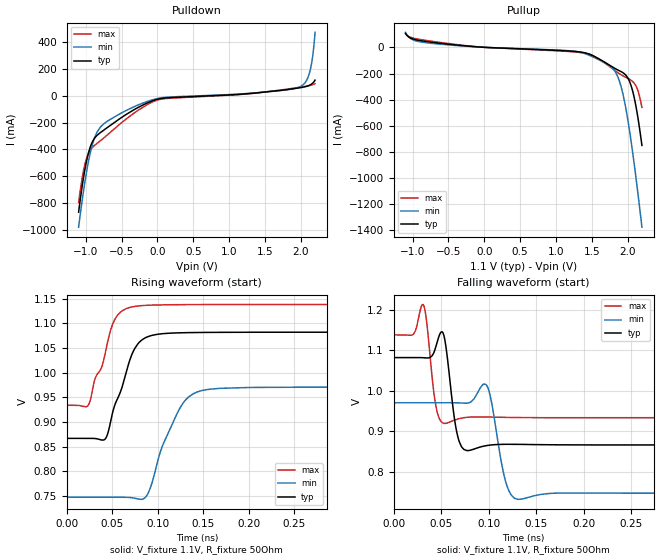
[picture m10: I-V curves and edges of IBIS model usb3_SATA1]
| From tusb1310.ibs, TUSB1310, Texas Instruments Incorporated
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|   USB 3.0 SATA1 mode, for SSTXP/N pin 750MHz
[Model]   usb3_SATA1
Model_type   Output
Polarity   Inverting
Vmeas = 0.96V
Vref = 1.1
Rref = 50
|   typ   min   max
|   (nom PVT)   (Fast PVT)   (slow PVT)
C_comp   0.5348pF   0.5225pF   0.5522pF
[Voltage Range]   1.1   0.99   1.155
[Temperature Range]   27   105   -40
[Pullup Reference]   1.1   0.99   1.155
[Pulldown Reference]   0   0   0
[Power Clamp Reference]   1.1   0.99   1.155
[GND Clamp Reference]   0   0   0
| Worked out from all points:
|   slope of the pulldown table from 0 to 0.165 V, typ, clamps not added: 14 ohm
|   slope of the pullup table from 0 to 0.165 V, typ, clamps not added: 40 ohm
|   falling waveform, V_fixture 1.1V, R_fixture 50Ohm: 20-80 % time 6.91ps typ, 9.83ps min, 5.71ps max; typ from 1.08 V to 0.867 V
|   rising waveform, V_fixture 1.1V, R_fixture 50Ohm: 20-80 % time 22.8ps typ, 27.8ps min, 20.9ps max; typ from 0.867 V to 1.08 V
[Pulldown]
|   Voltage   I(typ)   I(min)   I(max)
-1.1V     -868.9mA   -981.1mA   -796.9mA
-1.026V   -591.5mA   -690mA     -543.5mA
-951.1mV  -405.4mA   -461.1mA   -416.4mA
-868.4mV  -309.8mA   -301.2mA   -365.6mA
-744.4mV  -253.7mA   -206.5mA   -312.2mA
-297.7mV  -94.05mA   -73.91mA   -117.4mA
24.81mV   -21.49mA   -16.51mA   -26.68mA
1.977V    60.53mA    65.43mA    65.05mA
2.059V    68.81mA    98.55mA    72.03mA
2.117V    78.81mA    163.5mA    77.89mA
2.167V    95.9mA     297.7mA    84.86mA
2.2V      118.6mA    476.1mA    91.68mA
[Pullup]
|   Voltage   I(typ)   I(min)   I(max)
-1.1V     108.7mA    115.9mA    105.4mA
-992.5mV  63.95mA    57.32mA    71.65mA
-760.9mV  41.82mA    32.99mA    49.68mA
-16.54mV  1.455mA    1.316mA    1.593mA
1.406V    -41.39mA   -47.96mA   -43.61mA
1.77V     -143.3mA   -149.8mA   -155mA
1.877V    -176.7mA   -245mA     -198.4mA
1.968V    -208.9mA   -446.3mA   -227.1mA
2.026V    -260.1mA   -635.7mA   -243.8mA
2.084V    -364.9mA   -860.9mA   -269.2mA
2.142V    -532.4mA   -1.111A    -328.4mA
2.2V      -751.7mA   -1.378A    -460mA
[Ramp]
R_load = 50
|   typ   min   max
dV/dt_r   0.129193/2.27921e-11   0.134045/2.77619e-11   0.1226/2.09021e-11
dV/dt_f   0.129208/6.91542e-12   0.134061/9.83104e-12   0.122619/5.70782e-12
[Falling Waveform]
V_fixture = 1.1V
V_fixture_min = 0.99V
V_fixture_max = 1.155V
R_fixture = 50Ohm
C_fixture = 0F
|   Time   V(typ)   V(min)   V(max)
0s        1.082V     970.8mV    1.138V
32ps      1.082V     970.8mV    1.209V
44ps      1.106V     970.8mV    969.3mV
53ps      1.136V     970.8mV    920mV
66ps      904mV      970.7mV    929.5mV
77ps      852.9mV    969.8mV    934.7mV
99ps      865.5mV    1.009V     935.6mV
117ps     868.3mV    785mV      934.8mV
130ps     868.2mV    733.1mV    934.3mV
471ps     866.8mV    747.3mV    934mV
[Rising Waveform]
V_fixture = 1.1V
V_fixture_min = 0.99V
V_fixture_max = 1.155V
R_fixture = 50Ohm
C_fixture = 0F
|   Time   V(typ)   V(min)   V(max)
0s        866.8mV    747.4mV    934mV
23ps      866.8mV    747.4mV    932.5mV
42ps      865mV      747.4mV    1.037V
53ps      935.3mV    747.3mV    1.109V
71ps      1.034V     746.5mV    1.133V
88ps      1.072V     750.8mV    1.137V
105ps     1.079V     850.3mV    1.138V
123ps     1.081V     923.4mV    1.138V
147ps     1.082V     963mV      1.138V
471ps     1.082V     970.8mV    1.138V
